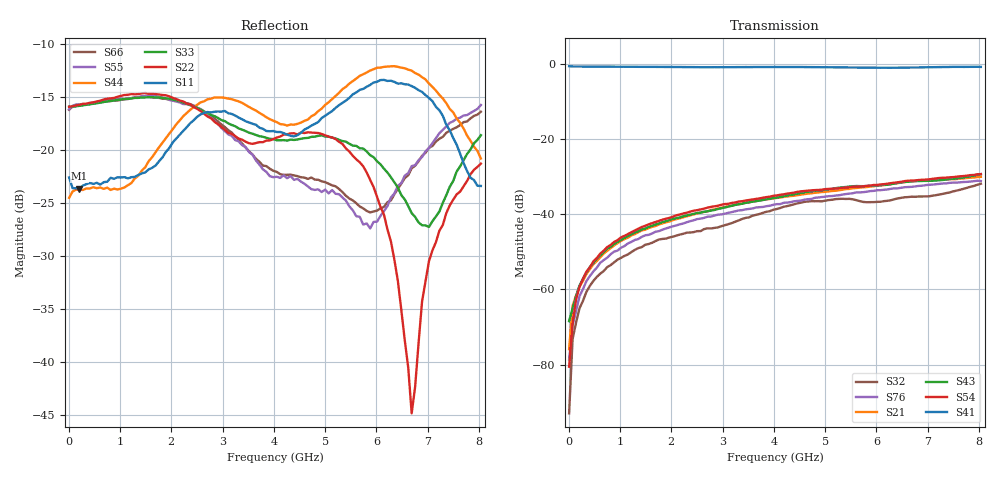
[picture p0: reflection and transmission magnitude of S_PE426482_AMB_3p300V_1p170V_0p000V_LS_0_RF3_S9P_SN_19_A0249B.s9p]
! Device ID: PE426482
! File Path: z:\PE426482\Final Char Data\room\AMB\3p300\LS_0_RF3\PE426482_AMB_3p300V_1p170V_0p000V_LS_0_RF3_S9P_SN_19_A0249B.s9p
! Serial: 19
! Lot: A0249B
! Temp: AMB
! VDD: 3.300
! VSS: 0.000
! Control_Hi: 1.170
! Control_Lo: 0.000
! Logic State: LS_0_RF3
! Port 1:
! Port 2:
! Port 3:
! Port 4:
! Port 5:
! Port 6:
! Port 7:
! Port 8:
! Port 9:
! ThroughPath:1-4
! IDD: 0.0001074886
! ISS/IDD2: 6.19e-008
! IDMM3/IDD3: -2.509e-007
! Comment:
#  Hz  S  RI  R  50
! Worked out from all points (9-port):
!   120 points, 10 MHz to 8.037 GHz, reference 50 ohm
!   strongest paths, dB at 10 MHz, 2.034 GHz, 4.057 GHz, 6.08 GHz, 8.037 GHz:
!     S41: -0.7, -0.9, -0.9, -1.1, -0.9
!     S54: -80.5, -40.7, -35.0, -32.1, -29.4
!     S43: -68.4, -41.3, -35.6, -32.3, -29.4
!     S21: -75.9, -41.6, -35.7, -32.4, -30.1
!     S76: -78.7, -43.2, -37.3, -33.6, -31.2
!     S32: -92.9, -46.0, -38.6, -36.7, -31.9
!   lowest |S11| = -23.7 dB at 212.3 MHz (marker M1), VSWR 1.14, Z = 57 - j0.526 ohm
!   |S11| at or under -10 dB: start of sweep to end of sweep
